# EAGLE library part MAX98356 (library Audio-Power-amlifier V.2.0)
The MAX98356 is a digital pulse-density modulated (PDM) input Class D power amplifier that provides Class AB audio performance with Class D efficiency. This IC offers five selectable gain settings (3dB, 6dB, 9dB, 12dB, and 15dB) set by a single gain-select input (GAIN).
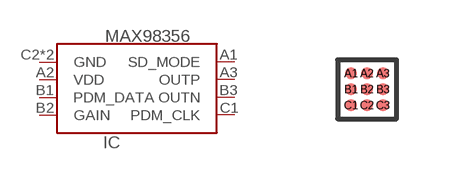
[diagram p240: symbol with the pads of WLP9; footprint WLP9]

Designator prefix IC

## MAX98356  [WLP9]
A1  SD_MODE
A2  VDD  pwr
A3  OUTP  out
B1  PDM_DATA  in
B2  GAIN
B3  OUTN  out
C1  PDM_CLK  in
C2  GND  pwr
C3  GND  pwr

## Footprint WLP9 (pad centres in mm)
WLP9 PACKAGE CODE BGA W91F1+1 www.maxim-ic.com/packages
smd 0.3 x 0.3: A1 -0.4,0.4; A2 0,0.4; A3 0.4,0.4; B1 -0.4,0; B2 0,0; B3 0.4,0; C1 -0.4,-0.4; C2 0,-0.4; C3 0.4,-0.4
